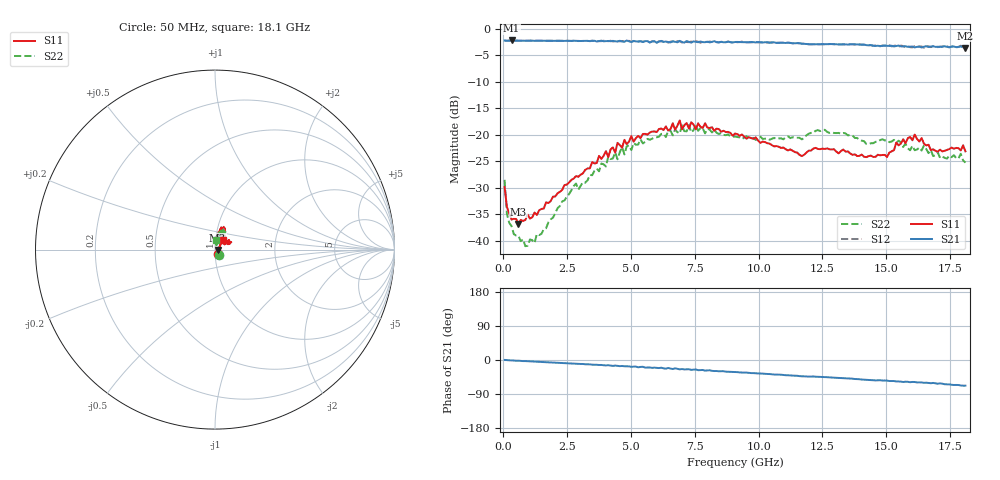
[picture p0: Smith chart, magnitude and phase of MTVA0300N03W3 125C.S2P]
! Network Analyzer HP8720D.06.14 Serial No. US36140669
!  7 Jul 2005  08:43:01
! Frequency  S11  S21  S12  S22
# HZ  S  DB R 50
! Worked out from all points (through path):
!   201 points, 50 MHz to 18.1 GHz, reference 50 ohm
!   highest |S21| = -2.24 dB at 320.8 MHz (marker M1); lowest = -3.7 dB at 18.1 GHz (marker M2)
!   group delay of S21, straight-line fit = 10.3 ps
!   lowest |S11| = -36.9 dB at 591.5 MHz (marker M3), VSWR 1.03, Z = 51.4 - j0.159 ohm
!   |S11| at or under -10 dB: start of sweep to end of sweep
!   |S22| runs from -41.1 to -18.2 dB; largest |S21 - S12| = 0.029
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5e7  -29.89 -53.2  -2.24 0.2  -2.26 0.2  -28.54 -50.2
1.4025e8  -33.67 -37.2  -2.31 -0.3  -2.29 -0.4  -34.98 -43.7
3.2075e8  -36.04 -19.3  -2.24 -1.0  -2.26 -0.9  -37.26 -25.4
5.915e8  -36.86 -6.2  -2.26 -1.9  -2.29 -2.0  -39.12 -4.2
1.22325e9  -34.71 13.3  -2.30 -4.3  -2.29 -4.3  -40.46 23.9
3.1185e9  -27.31 46.2  -2.32 -10.5  -2.35 -10.8  -28.97 79.0
4.021e9  -23.14 54.5  -2.36 -14.3  -2.37 -13.7  -26.03 76.5
4.11125e9  -24.25 54.7  -2.33 -13.7  -2.37 -14.5  -24.09 76.8
4.47225e9  -21.57 53.4  -2.44 -15.5  -2.33 -15.0  -24.68 81.2
4.65275e9  -22.48 54.2  -2.43 -15.8  -2.34 -16.5  -22.35 80.5
4.743e9  -21.00 58.2  -2.48 -16.6  -2.42 -16.0  -23.75 76.4
6.09675e9  -18.94 63.4  -2.46 -21.3  -2.37 -21.2  -20.40 70.7
6.909e9  -17.33 69.0  -2.31 -24.7  -2.39 -23.5  -19.79 65.7
6.99925e9  -19.01 68.0  -2.52 -23.8  -2.63 -25.3  -18.25 66.8
7.54075e9  -19.00 67.4  -2.49 -25.0  -2.37 -27.0  -18.18 68.8
9.075e9  -19.81 75.9  -2.53 -31.7  -2.51 -31.8  -20.38 58.5
1.169225e10  -24.06 65.1  -2.84 -43.1  -2.83 -42.9  -20.90 68.8
1.21435e10  -22.64 62.4  -2.96 -43.5  -2.92 -43.7  -19.60 72.8
1.512175e10  -23.40 35.4  -3.26 -55.5  -3.15 -55.1  -21.44 80.0
1.61145e10  -20.01 24.4  -3.56 -58.0  -3.31 -58.5  -22.95 71.9
1.674625e10  -22.93 27.9  -3.39 -61.3  -3.50 -61.5  -22.93 69.1
1.81e10  -23.16 50.4  -3.66 -67.7  -3.71 -68.6  -25.29 86.8
